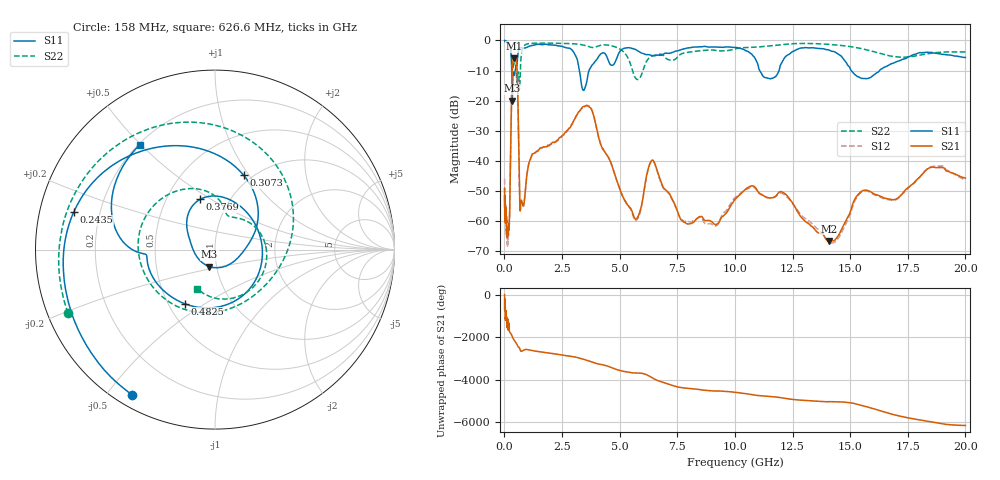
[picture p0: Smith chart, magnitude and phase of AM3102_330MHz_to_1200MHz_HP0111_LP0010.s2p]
! Date/Time: Tue, Sep 11, 2018 5:15 PM
! Network Analyzer: Agilent Technologies E8362B Rev: A.07.50.63
! Sweep from 0.010 to 20.000 GHz, 1601 Points, Sweep Type: LOG
! Power Supply: 4.949 V, 0.001 A
# Hz S DB R 50
!freq MagS11 AngS11 MagS21 AngS21 MagS12 AngS12 MagS22 AngS22
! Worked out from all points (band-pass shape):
!   1601 points, 10 MHz to 20 GHz, reference 50 ohm
!   highest |S21| = -5.96 dB at 432.6 MHz (marker M1); lowest = -66.8 dB at 14.07 GHz (marker M2)
!   |S21| within 3 dB of the highest: 346.7 MHz to 543.7 MHz (197 MHz wide, 44.3 % of centre)
!   lowest |S11| = -20.0 dB at 341.1 MHz (marker M3), VSWR 1.22, Z = 46.2 - j8.83 ohm
!   |S11| at or under -10 dB: 3.252 GHz to 3.673 GHz (420.6 MHz wide, 12.1 % of centre); 11.08 GHz to 11.92 GHz (841.3 MHz wide, 7.32 % of centre); 15.04 GHz to 16.28 GHz (1.235 GHz wide, 7.89 % of centre)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
!   |S22| runs from -16.2 to -0.2 dB; largest |S21 - S12| = 0.0073
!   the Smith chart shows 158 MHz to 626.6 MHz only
!   S11 on the Smith chart (normalised r, x): 158 MHz: 0.05, -0.58; 243.5 MHz: 0.10, +0.13; 307.3 MHz: 0.91, +0.94; 376.9 MHz: 0.73, +0.45; 482.5 MHz: 0.61, -0.42; 626.6 MHz: 0.21, +0.50
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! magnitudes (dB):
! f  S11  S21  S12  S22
! 10 MHz  0.0  -49.4  -46.1  -0.2
! 35.55 MHz  0.0  -60.1  -57.8  -0.4
! 126.4 MHz  -0.4  -64.6  -65.2  -0.8
! 158 MHz  -0.6  -64.6  -65.6  -1.0
! 243.5 MHz  -1.8  -50.8  -50.8  -1.9
! 307.3 MHz  -7.0  -19.8  -19.8  -4.8
! 341.1 MHz  -20.0  -9.8  -9.8  -8.8
! 376.9 MHz  -10.7  -6.9  -6.9  -9.0
! 432.6 MHz  -11.4  -6.0  -6.0  -7.4
! 447.2 MHz  -10.7  -6.0  -6.0  -7.3
! 482.5 MHz  -9.2  -6.2  -6.3  -8.0
! 559.1 MHz  -7.1  -11.4  -11.6  -13.5
! 626.6 MHz  -2.9  -36.7  -36.7  -12.4
! 692.3 MHz  -2.4  -56.6  -56.2  -10.5
! 1.59 GHz  -1.4  -35.7  -35.8  -0.9
! 3.651 GHz  -10.5  -22.0  -21.7  -2.0
! 5.652 GHz  -2.9  -59.3  -59.8  -12.1
! 6.426 GHz  -5.1  -39.8  -40.2  -5.1
! 7.882 GHz  -2.6  -60.9  -60.2  -4.0
! 10.73 GHz  -4.6  -48.4  -48.7  -2.3
! 14.07 GHz  -3.2  -66.8  -67.0  -1.3
! 20 GHz  -5.7  -45.8  -46.6  -3.8
